PROGRAM MAIN
VAR
	// 信号发生器
	ton1:Tc2_Standard.TON;
	// Json功能块
	jsonobj:JsonObjV5;
	// 时间采集
	gettime:Tc2_Utilities.NT_GetTime;
	
	// 数据库功能块
	fbNoSQLQueryBuilder_DocumentDB: FB_NoSQLQueryBuilder_DocumentDB;
	// 数据库请求命令
	fbNoSqlQuery : FB_NoSQLQueryEvt(sNetID := '', tTimeout := T#5S);
	// 数据库返回值
	fbNoSqlResult : FB_NoSQLResultEvt(sNetID := '', tTimeout := T#5S);
	// 数据插入
	InsertQueryOptions : Tc3_Database.T_QueryOptionDocumentDB_Insert;
	// 数据查询
	FindQueryOptions : Tc3_Database.T_QueryOptionDocumentDB_Find;
	// 数据查找
	datasearch : STRING(1000) := '{eventdiscription : "too large"}';
	// 查询返回，默认返回20个数据
	dataDocument : ARRAY[1..20] OF STRING(1000);
	// 返回信息
	InfoResult: Tc3_Database.I_TcMessage;
	
	// 数据
	demodata:demoDUT;
	// 转化的json对象
	jsondata:STRING(1000);
	// 查询异常数据
	read:BOOL;
END_VAR

// 调用信号发生器
SigGen();
// 读取系统时间
fbgettime();
// 数据赋值
setData();
// 结构体转化为json字符串
jsondata:=jsonobj.ObjToJsonStr(nData:= SIZEOF(demodata), pData:= ADR(demodata));
// 信号触发之后保存数据
IF ton1.Q THEN
	SaveData();
END_IF
// 查询
IF read THEN
	ReadData();
END_IF

ACTION fbgettime:
gettime(
	NETID:= '', 
	START:= ton1.Q, 
	TMOUT:= , 
	BUSY=> , 
	ERR=> , 
	ERRID=> , 
	TIMESTR=> demodata.timedata);
END_ACTION

ACTION ReadData:
FindQueryOptions.pFilter:= ADR(datasearch);
FindQueryOptions.cbFilter:= SIZEOF(datasearch); 

fbNoSQLQueryBuilder_DocumentDB.eQueryType := Tc3_Database.E_DocumentDbQueryType.Find;
fbNoSQLQueryBuilder_DocumentDB.sCollectionName := 'twincat';
fbNoSQLQueryBuilder_DocumentDB.pQueryOptions := ADR(FindQueryOptions);
fbNoSQLQueryBuilder_DocumentDB.cbQueryOptions := SIZEOF(FindQueryOptions);

IF fbNoSqlQuery.ExecuteDataReturn(hDBID:= 2, iNoSQLQueryBuilder:= fbNoSQLQueryBuilder_DocumentDB, pNoSQLResult:= ADR(fbNoSqlResult)) THEN
	IF fbNoSqlQuery.bError THEN
		InfoResult := fbNoSqlQuery.ipTcResult;
	ELSE
		IF fbNoSqlResult.ReadAsString(nStartIndex:= 0, nRecordCount:= 20, pData:= ADR(dataDocument), cbData:= SIZEOF(dataDocument), 
			MaxDocumentSize:= SIZEOF(dataDocument[1]), bDataRelease:= TRUE) THEN
			IF fbNoSqlResult.bError THEN
				InfoResult := fbNoSqlResult.ipTcResult;
			END_IF
		END_IF
	END_IF
END_IF
END_ACTION

ACTION SaveData:
InsertQueryOptions.pDocuments:= ADR(jsondata); 
InsertQueryOptions.cbDocuments:= SIZEOF(jsondata);

fbNoSQLQueryBuilder_DocumentDB.eQueryType := E_DocumentDbQueryType.InsertOne;
fbNoSQLQueryBuilder_DocumentDB.sCollectionName := 'twincat';
fbNoSQLQueryBuilder_DocumentDB.pQueryOptions := ADR(InsertQueryOptions);
fbNoSQLQueryBuilder_DocumentDB.cbQueryOptions := SIZEOF(InsertQueryOptions);

IF fbNoSQLQuery.Execute(2, fbNoSQLQueryBuilder_DocumentDB) THEN
	IF fbNoSQLQuery.bError THEN
		InfoResult := fbNoSQLQuery.ipTcResult;
	END_IF
END_IF
END_ACTION

ACTION setData:
// 采样记录的时间
demodata.timedata:=gettime.TIMESTR;
// 采样数据
demodata.realdata:=demoDataGen.dataout;
// 判断数据是否异常，加入描述
IF (demodata.realdata > 0.7) THEN
	demodata.eventdiscription:='too large';
ELSE
	demodata.eventdiscription:='normal state';
END_IF
END_ACTION

ACTION SigGen:
// 采样信号发生器
ton1(IN:= NOT ton1.Q, PT:= t#3s, Q=> , ET=> );
END_ACTION

END_PROGRAM
